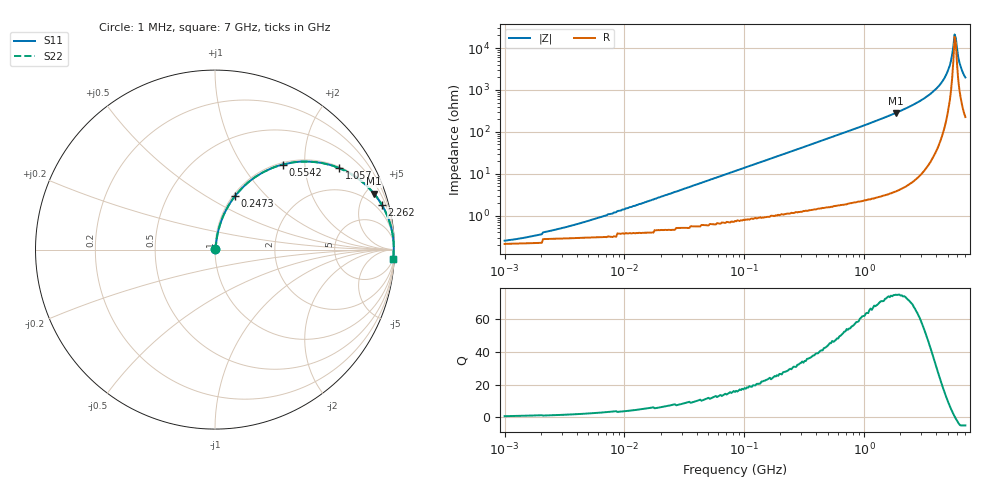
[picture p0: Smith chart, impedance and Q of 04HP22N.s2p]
# MHz S MA R 50
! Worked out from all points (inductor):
!   385 points, 1 MHz to 7 GHz, reference 50 ohm
!   read as one part in series: L = 22 nH near 6.778 MHz
!   highest Q = 74.7 at 1.838 GHz (marker M1), where L = 24.5 nH
!   self-resonance near 5.688 GHz
!   S11 on the Smith chart (normalised r, x): 1 MHz: 1.00, +0.00; 247.3 MHz: 1.02, +0.69; 554.2 MHz: 1.03, +1.55; 1.057 GHz: 1.05, +3.02; 2.262 GHz: 1.10, +7.40; 7 GHz: 5, -39
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1  0.002616 31.7  0.998 -0.1  0.998 -0.1  0.002616 31.7
2.044  0.003761 48.4  0.998 -0.2  0.998 -0.2  0.003761 48.4
4.374  0.006692 63.9  0.997 -0.3  0.997 -0.3  0.006692 63.9
19.575  0.027 79.3  0.995 -1.5  0.995 -1.5  0.027 79.3
85.617  0.117 79.7  0.986 -6.7  0.986 -6.7  0.117 79.7
247.271  0.321 69.4  0.936 -18.7  0.936 -18.7  0.321 69.4
365.931  0.448 61.8  0.882 -26.6  0.882 -26.6  0.448 61.8
554.163  0.605 51.5  0.783 -37.3  0.783 -37.3  0.605 51.5
1056.84  0.828 33.2  0.548 -55.9  0.548 -55.9  0.828 33.2
1637.803  0.922 22.0  0.374 -67.3  0.374 -67.3  0.922 22.0
1837.926  0.939 19.4  0.332 -69.9  0.332 -69.9  0.939 19.4
2261.765  0.962 15.1  0.26 -74.2  0.26 -74.2  0.962 15.1
3586.848  0.99 7.0  0.122 -81.7  0.122 -81.7  0.99 7.0
4516.955  0.995 3.5  0.061 -83.5  0.061 -83.5  0.995 3.5
5187.11  0.996 1.5  0.026 -80.2  0.026 -80.2  0.996 1.5
5431.903  0.996 0.8  0.014 -73.2  0.014 -73.2  0.996 0.8
5558.598  0.996 0.5  0.008934 -62.5  0.008934 -62.5  0.996 0.5
5688.248  0.996 0.1  0.004717 -27.3  0.004717 -27.3  0.996 0.1
5820.923  0.996 -0.2  0.005635 39.7  0.005635 39.7  0.996 -0.2
6095.627  0.995 -0.9  0.016 72.2  0.016 72.2  0.995 -0.9
6237.803  0.995 -1.2  0.022 76.0  0.022 76.0  0.995 -1.2
7000  0.993 -2.9  0.05 80.6  0.05 80.6  0.993 -2.9
